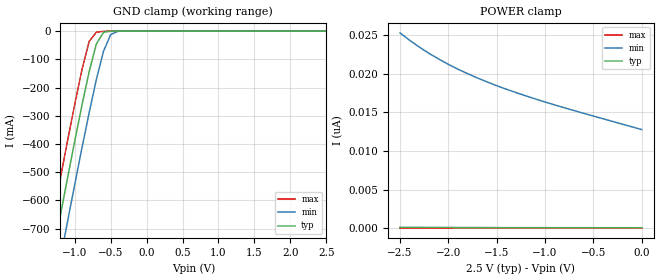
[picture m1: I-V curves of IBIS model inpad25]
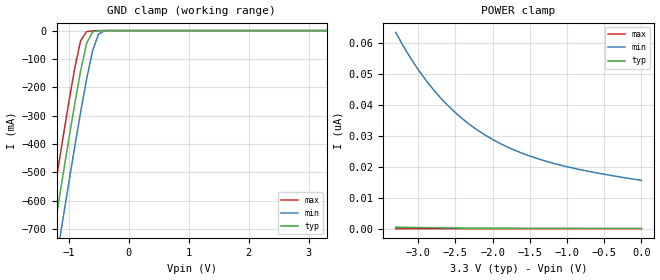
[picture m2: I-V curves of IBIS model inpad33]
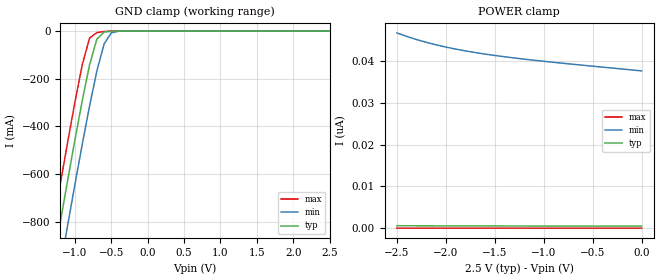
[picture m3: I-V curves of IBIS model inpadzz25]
| IBIS file abc.ibs created by s2ibis2 version 1.2
| North Carolina State University Electronics Research Laboratory  1995
[IBIS ver]   2.1
[File name]   idt70t6xx_144dd.ibs
[File Rev]   1.0
[Date]   12/19/2002
[Source]   Integrated Device Technology, Inc.
[Notes]   1.Temperatures: typ=25C, min=100C, max=0C 2.RRmp rates based
   on 50 ohm load.
[Disclaimer] Integrated Device Technology, Inc. ("IDT") hereby grants the
   user of this IBIS model a non-exclusive, nontransferable
   license to use this IBIS model under the following terms. The
   user is granted this license only to use the IBIS model and is
   not granted rights to sell, copy (except as needed to run the
   IBIS model), rent, lease or sub-license the IBIS model in
   whole or in part, or in modified form to anyone. The User may
   modify the IBIS model to suit its specific applications, but
   rights to derivative works and such modifications shall belong
   to IDT. This IBIS model is provided on an AS IS" basis and IDT
   makes absolutely no warranty with respect to the information
   contained herein. IDT DISCLAIMS AND CUSTOMER WAIVES ALL
   WARRANTIES, EXPRESS AND IMPLIED, INCLUDING WARRANTIES OF
   MERCHANTABILITY AND FITNESS FOR A PARTICULAR PURPOSE. THE
   ENTIRE RISK AS TO QUALITY AND PERFORMANCE IS WITH THE USER
   ACCORDINGLY, IN NO EVENT SHALL IDT BE LIABLE FOR ANY DIRECT OR
   INDIRECT DAMAGES, WHETHER IN CONTRACT OR TORT, INCLUDING ANY
   LOST PROFITS OR OTHER INCIDENTAL, CONSEQUENTIAL, EXEMPLARY, OR
   PUNITIVE DAMAGES ARISING OUT OF THE USE OR APPLICATION OF THE
   IBIS model. Further, IDT reserves the right to make changes
   without notice to any product herein to improve reliability,
   function, or design. IDT does not convey any license under
   patent rights or any other intellectual property rights,
   including those of third parties. IDT is not obligated to
   provide maintenance or support for the licensed IBIS model.
[Copyright]   Copyright 2001, Integrated Device Technology, Inc. all rights
   reserved
|   Component idt70t6xx_144dd
[Component]   idt70t6xx_144dd
[Manufacturer]   Integrated Device Technology
[Package]
| variable   typ   min   max
R_pkg   0.19600   0.19500   0.196000
L_pkg   13.1000nH   10.8200nH   15.36000nH
C_pkg   1.92000pF   1.90000pF   1.940000pF
| NOTE:
| The model_name inpad, inpadzz, and iopad work for both 3.3v and 2.5v
| vddq.  When vddq is 3.3v, the model names are inpad33, inpadzz33, and
| iopad33.  When vddq is 2.5v, the model names will be inpad25, inpadzz25,
| and iopad25.  This package does not have JTAG features.
[Pin]  signal_name   model_name   R_pin   L_pin   C_pin
1   vss/test   GND
2   vddqr   POWER
3   vss   GND
4   vddql   POWER
5   vss   GND
6   vddqr   POWER
7   vss   GND
8   io5l   iopad25
9   io5r   iopad25
10   vddql   POWER
11   vss   GND
12   io6l   iopad25
13   io6r   iopad25
14   vddqr   POWER
15   zzr   inpadzz25
16   vdd   POWER
17   vdd   POWER
18   vss   GND
19   vss   GND
20   vddql   POWER
21   vss   GND
22   io7r   iopad25
23   io7l   iopad25
24   io8r   iopad25
25   io8l   iopad25
26   vddqr   POWER
27   vss   GND
30   vddql   POWER
31   vss   GND
32   vddqr   POWER
33   vss   GND
34   vss   GND
35   vddql   POWER
37   vdd   POWER
40   a18r   inpad25
41   a17r   inpad25
42   a16r   inpad25
43   a15r   inpad25
44   a14r   inpad25
45   a13r   inpad25
46   a12r   inpad25
47   a11r   inpad25
48   a10r   inpad25
49   a9r   inpad25
50   a8r   inpad25
51   a7r   inpad25
54   ce1r   inpad25
55   ce0rb   inpad25
56   vdd   POWER
57   vss   GND
58   semrb   inpad25
59   oerb   inpad25
60   rwr   inpad25
61   busyrb   iopad25
62   intrb   iopad25
63   msb   inpad25
64   a6r   inpad25
65   a5r   inpad25
66   a4r   inpad25
67   a3r   inpad25
68   a2r   inpad25
69   a1r   inpad25
70   a0r   inpad25
71   vdd   POWER
72   vss   GND
73   optr   inpad25
74   vddql   POWER
75   vss   GND
76   vddqr   POWER
77   vss   GND
78   vddql   POWER
79   vss   GND
80   io0l   iopad25
81   io0r   iopad25
82   vddqr   POWER
83   vss   GND
84   io1l   iopad25
85   io1r   iopad25
86   io2l   iopad25
87   io2r   iopad25
88   vddql   POWER
89   zzl   inpadzz25
90   vss   GND
91   vss   GND
92   vdd   POWER
93   vdd   POWER
94   vddqr   POWER
95   vss   GND
96   io3r   iopad25
97   io3l   iopad25
98   vddql   POWER
99   vss   GND
100   io4r   iopad25
101   io4l   iopad25
102   vddqr   POWER
103   vss   GND
104   vddql   POWER
105   vss   GND
106   vss   GND
107   vddqr   POWER
108   optl   inpad25
109   vss   GND
110   vdd   POWER
111   a0l   inpad25
112   a1l   inpad25
113   a2l   inpad25
114   a3l   inpad25
115   a4l   inpad25
116   a5l   inpad25
117   a6l   inpad25
119   intlb   iopad25
120   busylb   iopad25
121   rwl   inpad25
122   oelb   inpad25
123   semlb   inpad25
124   vss   GND
125   vdd   POWER
126   ce0lb   inpad25
127   ce1l   inpad25
130   a7l   inpad25
131   a8l   inpad25
132   a9l   inpad25
133   a10l   inpad25
134   a11l   inpad25
135   a12l   inpad25
136   a13l   inpad25
137   a14l   inpad25
138   a15l   inpad25
139   a16l   inpad25
140   a17l   inpad25
141   a18l   inpad25
144   vdd   POWER
|in   in   dummy_model
|oe   oe   dummy_model
| needed to give pads seperate POWER supply
[Pin Mapping] pulldown_ref   pullup_ref
1   vss   nc
2   nc   vddqr
3   vss   nc
4   nc   vddql
5   vss   nc
6   nc   vddqr
7   vss   nc
8   vss   vddql
9   vss   vddqr
10   nc   vddql
11   vss   nc
12   vss   vddql
13   vss   vddqr
14   nc   vddqr
15   vss   vdd
16   nc   vdd
17   nc   vdd
18   vss   nc
19   vss   nc
20   nc   vddql
21   vss   nc
22   vss   vddqr
23   vss   vddql
24   vss   vddqr
25   vss   vddql
26   nc   vddqr
27   vss   nc
30   nc   vddql
31   vss   nc
32   nc   vddqr
33   vss   nc
34   vss   nc
35   nc   vddql
37   nc   vdd
40   vss   vdd
41   vss   vdd
42   vss   vdd
43   vss   vdd
44   vss   vdd
45   vss   vdd
46   vss   vdd
47   vss   vdd
48   vss   vdd
49   vss   vdd
50   vss   vdd
51   vss   vdd
54   vss   vdd
55   vss   vdd
56   nc   vdd
57   vss   nc
58   vss   vdd
59   vss   vdd
60   vss   vdd
61   vss   vddqr
62   vss   vddqr
63   vss   vdd
64   vss   vdd
65   vss   vdd
66   vss   vdd
67   vss   vdd
68   vss   vdd
69   vss   vdd
70   vss   vdd
71   nc   vdd
72   vss   nc
73   vss   vdd
74   nc   vddql
75   vss   nc
76   nc   vddqr
77   vss   nc
78   nc   vddql
79   vss   nc
80   vss   vddql
81   vss   vddqr
82   nc   vddqr
83   vss   nc
84   vss   vddql
85   vss   vddqr
86   vss   vddql
87   vss   vddqr
88   nc   vddql
89   vss   vdd
90   vss   nc
91   vss   nc
92   nc   vdd
93   nc   vdd
94   nc   vddqr
95   vss   nc
96   vss   vddqr
97   vss   vddql
98   nc   vddql
99   vss   nc
100   vss   vddqr
101   vss   vddql
102   nc   vddqr
103   vss   nc
104   nc   vddql
105   vss   nc
106   vss   nc
107   nc   vddqr
108   vss   vdd
109   vss   nc
110   nc   vdd
111   vss   vdd
112   vss   vdd
113   vss   vdd
114   vss   vdd
115   vss   vdd
116   vss   vdd
117   vss   vdd
119   vss   vddql
120   vss   vddql
121   vss   vdd
122   vss   vdd
123   vss   vdd
124   vss   nc
125   nc   vdd
126   vss   vdd
127   vss   vdd
130   vss   vdd
131   vss   vdd
132   vss   vdd
133   vss   vdd
134   vss   vdd
135   vss   vdd
136   vss   vdd
137   vss   vdd
138   vss   vdd
139   vss   vdd
140   vss   vdd
141   vss   vdd
144   nc   vdd
| Models and submodels in the file (6): inpad25 (Input), inpad33 (Input), inpadzz25 (Input), inpadzz33 (Input), iopad25 (I/O), iopad33 (I/O)
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|in   nc   nc
|oe   nc   nc
| Note:
| 1. Pins 40 and 141 are nc for idt70t631, and idt70t639.
| 2. Pins 41 and 140 are nc for idt70t639.
|   Model inpad25
[Model]   inpad25
Model_type   Input
Polarity   Non-Inverting
Vinl =  0.70000V
Vinh =  1.70000V
Vmeas =  1.25000V
C_comp   4.50000pF   4.50000pF   4.50000pF
[Temperature Range]   25.00000   100.00000   -40.00000
[Voltage Range]   2.50000V   2.30000V   2.70000V
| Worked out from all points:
|   GND clamp passes 1 mA (typ) near -0.52 V on its own axis
[GND_clamp]
| voltage   I(typ)   I(min)   I(max)
-2.5V     -2.438A    -2.587A    -2.312A
-1.4V     -921.5mA   -1.075A    -790.4mA
-1.3V     -786.2mA   -940.4mA   -654.7mA
-1.2V     -651.9mA   -806.3mA   -520.2mA
-1.1V     -519.1mA   -673.5mA   -387.5mA
-900mV    -262mA     -413.5mA   -136.1mA
-800mV    -143.3mA   -288.9mA   -36.33mA
-700mV    -45.49mA   -171.6mA   -3.972mA
-600mV    -4.309mA   -71.06mA   -834.5uA
-500mV    -411.8uA   -12.18mA   -82.9uA
-400mV    -35.7uA    -828.2uA   -3.321uA
2.5V      53.96pA    13.46nA    209.5fA
[POWER_clamp]
| voltage   I(typ)   I(min)   I(max)
-2.5V     115.4pA    25.27nA    455.8fA
-2.4V     107.8pA    24.31nA    438fA
-2.3V     101.2pA    23.43nA    421.7fA
-2.2V     95.32pA    22.62nA    405.4fA
-2.1V     90.21pA    21.89nA    391.5fA
-1.9V     81.83pA    20.57nA    366.6fA
-1.6V     72.81pA    18.93nA    335.5fA
-1.4V     68.5pA     17.98nA    318.8fA
-1V       62.48pA    16.33nA    288.4fA
-600mV    58.51pA    14.86nA    261.9fA
0V        53.96pA    12.76nA    222.8fA
|   Model inpad33
[Model]   inpad33
Model_type   Input
Polarity   Non-Inverting
Vinl =  0.80000V
Vinh =  2.00000V
Vmeas =  1.50000V
C_comp   4.50000pF   4.50000pF   4.50000pF
[Temperature Range]   25.00000   100.00000   -40.00000
[Voltage Range]   3.30000V   3.10000V   3.50000V
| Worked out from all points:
|   GND clamp passes 1 mA (typ) near -0.52 V on its own axis
[GND_clamp]
| voltage   I(typ)   I(min)   I(max)
-3.3V     -3.553A    -3.699A    -3.43A
-1.4V     -921.5mA   -1.075A    -790.4mA
-1.3V     -786.2mA   -940.4mA   -654.7mA
-1.2V     -651.9mA   -806.3mA   -520.2mA
-1.1V     -519.1mA   -673.5mA   -387.5mA
-900mV    -262mA     -413.5mA   -136.1mA
-800mV    -143.3mA   -288.9mA   -36.33mA
-700mV    -45.49mA   -171.6mA   -3.972mA
-600mV    -4.309mA   -71.06mA   -834.5uA
-500mV    -411.8uA   -12.18mA   -82.9uA
-400mV    -35.7uA    -828.2uA   -3.321uA
3.3V      60.32pA    16.33nA    261.7fA
[POWER_clamp]
| voltage   I(typ)   I(min)   I(max)
-3.3V     485.3pA    63.31nA    1.192pA
-3.2V     440.5pA    58.98nA    1.104pA
-3V       362.8pA    51.38nA    959fA
-2.9V     329.2pA    48.06nA    890.9fA
-2.7V     271.6pA    42.26nA    779.3fA
-2.4V     205pA      35.37nA    648fA
-2.1V     157.4pA    30.2nA     551.4fA
-1.9V     133.8pA    27.5nA     498.7fA
-1.7V     115.4pA    25.27nA    457.1fA
-1.3V     90.21pA    21.88nA    391.5fA
-700mV    70.52pA    18.44nA    327.3fA
0V        60.32pA    15.58nA    275.6fA
|   Model inpadzz25
[Model]   inpadzz25
Model_type   Input
Polarity   Non-Inverting
Vinl =  0.80000V
Vinh =  2.00000V
Vmeas =  1.50000V
C_comp   4.50000pF   4.50000pF   4.50000pF
[Temperature Range]   25.00000   100.00000   -40.00000
[Voltage Range]   2.50000V   2.20000V   2.80000V
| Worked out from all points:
|   GND clamp passes 1 mA (typ) near -0.51 V on its own axis
[GND_clamp]
| voltage   I(typ)   I(min)   I(max)
-2.5V     -3.145A    -3.326A    -2.992A
-1.4V     -1.152A    -1.34A     -992.6mA
-1.3V     -975mA     -1.163A    -814.5mA
-1.2V     -799.1mA   -987.7mA   -638.3mA
-1.1V     -625.5mA   -813.9mA   -465mA
-900mV    -292mA     -475.5mA   -141.4mA
-800mV    -142.5mA   -315.2mA   -29.66mA
-700mV    -33.97mA   -168.4mA   -6.415mA
-600mV    -4.291mA   -54.25mA   -1.765mA
-500mV    -767.5uA   -6.912mA   -190.3uA
-400mV    -75.7uA    -637.7uA   -8.282uA
2.5V      493.9pA    38.32nA    3.386pA
[POWER_clamp]
| voltage   I(typ)   I(min)   I(max)
-2.5V     588.9pA    46.73nA    4.616pA
-2.4V     578.8pA    45.89nA    4.553pA
-2.3V     569.9pA    45.14nA    4.503pA
-2.2V     562pA      44.48nA    4.452pA
-2.1V     555pA      43.88nA    4.404pA
-1.9V     543.3pA    42.86nA    4.294pA
-1.8V     538.5pA    42.42nA    4.255pA
-1.6V     530.2pA    41.66nA    4.162pA
-1.4V     523.5pA    41.02nA    4.079pA
-1.1V     515.4pA    40.19nA    3.956pA
-800mV    508.8pA    39.45nA    3.825pA
0V        493.9pA    37.64nA    3.507pA
